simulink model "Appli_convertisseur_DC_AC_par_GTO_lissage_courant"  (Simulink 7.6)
settings: Solver=ode23tb  StartTime=0.0  StopTime=2  RelTol=1e-3
InitFcn:
  | T=1/60;
StopFcn:
  | close all
  | load I_RL.mat
  | 
  | plot(x(1,:),x(2,:))
  | grid
  | axis([0 2 -11 11])
  | title('Courant dans la charge - bobine de lissage')
  | xlabel('temps')
libraries: powerlib x12

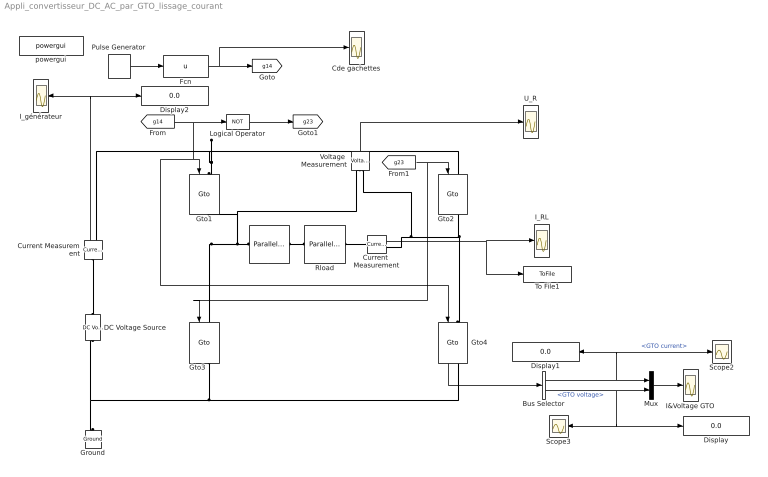
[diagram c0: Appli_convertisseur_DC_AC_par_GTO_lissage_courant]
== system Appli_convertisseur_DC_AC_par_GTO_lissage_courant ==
  Bus Selector : BusSelector  OutputSignals=GTO current,GTO voltage
  Cde gachettes : Scope
  Current  Measurement : powerlib/Measurements/Current Measurement  DialogController=POWERSYS.PowerSysDialog  SystemSampleTime=-1  PhasorSimulation=off  OutputType=Complex  PSBequivalent=0
  Current Measurement : powerlib/Measurements/Current Measurement  DialogController=POWERSYS.PowerSysDialog  SystemSampleTime=-1  PhasorSimulation=off  OutputType=Complex  PSBequivalent=0
  DC Voltage Source : powerlib/Electrical Sources/DC Voltage Source  DialogController=POWERSYS.PowerSysDialog  SystemSampleTime=-1  Amplitude=12  Measurements=None
  Display : Display
  Display1 : Display
  Display2 : Display
  Fcn : Fcn  Expr=u
  Ground : powerlib/Elements/Ground  DialogController=POWERSYS.PowerSysDialog  PhysicalDomain=powersysdomain  SubClassName=unknown  LeftPortType=p1  RightPortType=p1  LConnTagsString=a
  Gto{1..4} (4 alike) : powerlib/Power Electronics/Gto  DialogController=POWERSYS.PowerSysDialog  SystemSampleTime=-1  Ron=0.001  Lon=0  Vf=1  Tf=10e-6  Tt=20e-6  IC=0  Rs=1e5  Cs=inf  Measurements=on
  I&Voltage GTO : Scope
  I_RL : Scope
  I_générateur : Scope
  L : powerlib/Elements/Parallel RLC Branch  DialogController=POWERSYS.PowerSysDialog  PhysicalDomain=powersysdomain  SubClassName=unknown  LeftPortType=p1  RightPortType=p1  LConnTagsString=a  RConnTagsString=__new0  BranchType=L  Resistance=1  Inductance=0.1  SetiL0=off  InitialCurrent=0  Capacitance=1e-6  Setx0=off  InitialVoltage=0  Measurements=None
  Logical Operator : Logic  Operator=NOT  AllPortsSameDT=off  OutDataTypeStr=boolean
  Mux : Mux  Inputs=2
  Pulse Generator : DiscretePulseGenerator  PulseType=Time based  Period=1  PulseWidth=50
  Rload : powerlib/Elements/Parallel RLC Branch  DialogController=POWERSYS.PowerSysDialog  PhysicalDomain=powersysdomain  SubClassName=unknown  LeftPortType=p1  RightPortType=p1  LConnTagsString=a  RConnTagsString=__new0  BranchType=R  Resistance=1  Inductance=1e-3  SetiL0=off  InitialCurrent=0  Capacitance=1e-6  Setx0=off  InitialVoltage=0  Measurements=None
  Scope2 : Scope
  Scope3 : Scope
  To File1 : ToFile  Filename=I_RL  MatrixName=x
  U_R : Scope
  Voltage  Measurement : powerlib/Measurements/Voltage Measurement  DialogController=POWERSYS.PowerSysDialog  SystemSampleTime=-1  PhasorSimulation=off  OutputType=Complex  PSBequivalent=0
  powergui : powerlib/powergui  Priority=2  SystemSampleTime=-1  SimulationMode=Continuous  SampleTime=0  frequency=60  SPID=off  DisableSnubberDevices=off  DisableRonSwitches=off  DisableVfSwitches=off  SwTol=0  Interpol=off  frequencyindice=0  echomessages=off  HookPort=off  DisplayEquations=off  FunctionMessages=off  EnableUseOfTLC=off  x0status=blocks  RestoreLinks=warning  ResistiveCurrentMeasurement=off  Frange=logspace(0,3,50)  Ylog=off  Xlog=off  ShowGrid=off  save=off  variable=ZData  ZoomFFT=on  StartTime=0.0  cycles=1  DisplayStyle=off  fundamental=60  FreqAxis=off  MaxFrequency=1000  frequencyindicesteady=1  RmsSteady=1  display=off  Ts=0  methode=off
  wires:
  Voltage  Measurement/1 -> U_R/1
  [g14] -> Gto4/1, Gto1/1, Logical Operator/1
  [g23] -> Gto2/1, Gto3/1
  Logical Operator/1 -> [g23]
  Gto4/1 -> Bus Selector/1
  Bus Selector/1 -> Mux/1, Display1/1, Scope2/1  "<GTO current>"
  Bus Selector/2 -> Mux/2, Display/1, Scope3/1  "<GTO voltage>"
  Mux/1 -> I&Voltage GTO/1
  Current Measurement/1 -> I_générateur/1, Display2/1
  Current  Measurement/1 -> I_RL/1, To File1/1
  Pulse Generator/1 -> Fcn/1
  Fcn/1 -> [g14], Cde gachettes/1
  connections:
  Gto3/RConn1 -- Ground/LConn1 -- DC Voltage Source/LConn1 -- Gto4/RConn1
  Voltage  Measurement/LConn2 -- Gto4/LConn1 -- Gto2/RConn1 -- Current  Measurement/RConn1
  Gto1/LConn1 -- Current Measurement/RConn1 -- Gto2/LConn1
  Current Measurement/LConn1 -- DC Voltage Source/RConn1
  L/RConn1 -- Rload/LConn1
  Current  Measurement/LConn1 -- Rload/RConn1
  Gto3/LConn1 -- Gto1/RConn1 -- L/LConn1 -- Voltage  Measurement/LConn1
